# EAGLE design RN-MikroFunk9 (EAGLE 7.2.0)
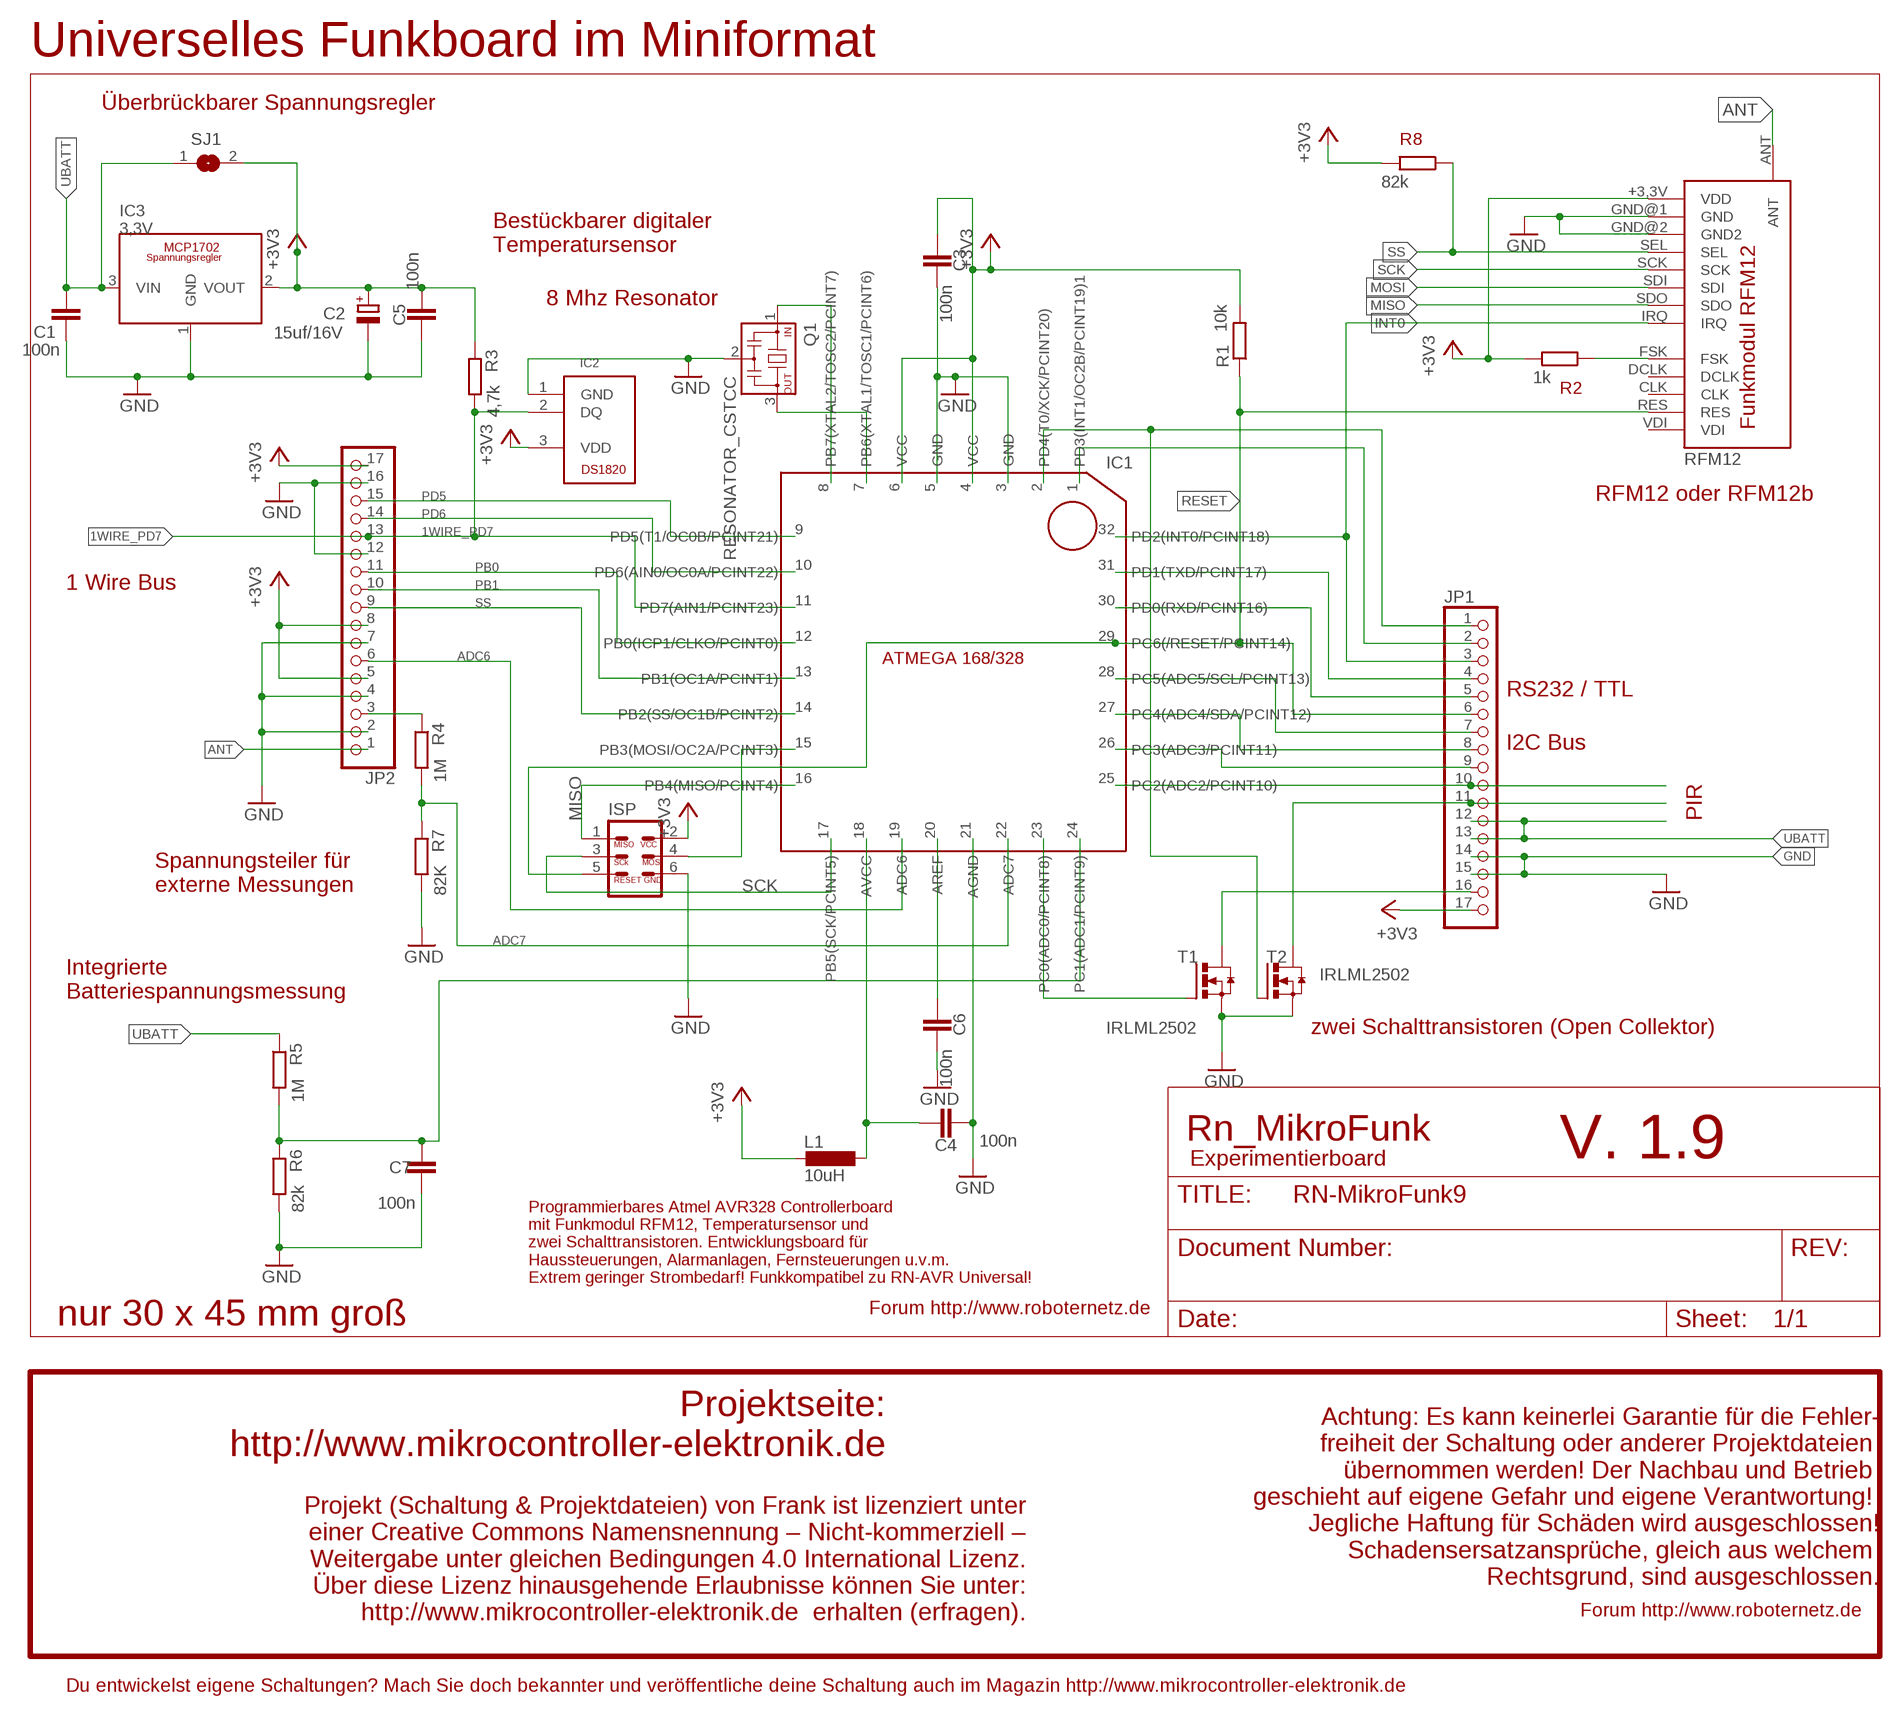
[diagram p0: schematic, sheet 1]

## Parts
C1  100n  C-EUC1206  [C1206]
C2  15uf/16V  CPOL-EUSMCC  [SMC_C]
C3  100n  C-EUC1206  [C1206]
C4  100n  C-EUC1206  [C1206]
C5  100n  C-EUC1206  [C1206]
C6  100n  C-EUC1206  [C1206]
C7  100n  C-EUC1206  [C1206]
IC1  ATMEGA168/328_SMD_PINANSICHT  [TQFP32-08]
IC2  DS1820  [TO92-]
IC3  3,3V  MCP1702SOT23  [SOT23]
ISP  ISP6  [ISP6DICK]
JP1  PINHD-1X17  [1X17]
JP2  PINHD-1X17  [1X17]
L1  10uH  L-SMD-1206  [L1206]
Q1  RESONATOR_CSTCC  [RESONATOR_CSTCC]
R1  10k  R-EU_M1206  [M1206]
R2  1k  R-EU_M1206  [M1206]
R3  4,7k  R-EU_M1206  [M1206]
R4  1M  R-EU_M1206  [M1206]
R5  1M  R-EU_M1206  [M1206]
R6  82k  R-EU_M1206  [M1206]
R7  82K  R-EU_M1206  [M1206]
R8  82k  R-EU_M1206  [M1206]
RFM12  RFM12  [RFM12_SMD]
SJ1  SJ  [SJ]
T1  IRLML2502  [MICRO3]
T2  IRLML2502  [MICRO3]

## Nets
1WIRE_PD7: IC1.11(PD7(AIN1/PCINT23)) IC2.2(DQ) JP2.13 R3.2
+3V3 [Power]: C2.+ C3.2 C5.1 IC1.4(VCC) IC1.6(VCC) IC2.3(VDD) IC3.2(VOUT) ISP.2 JP1.17 JP2.5 JP2.8 JP2.17 L1.2 R1.2 R2.2 R3.1 R8.2 RFM12.+3,3V(VDD) SJ1.2
ADC2: IC1.25(PC2(ADC2/PCINT10)) JP1.10
ADC3: IC1.26(PC3(ADC3/PCINT11)) JP1.9
ADC4: IC1.27(PC4(ADC4/SDA/PCINT12)) JP1.8
ADC5: IC1.28(PC5(ADC5/SCL/PCINT13)) JP1.7
ADC6: IC1.19(ADC6) JP2.6
ADC7: IC1.22(ADC7) R4.2 R7.1
ANT: JP2.1 RFM12.ANT
GND [Power]: C1.1 C2.- C3.1 C4.1 C5.2 C6.1 C7.1 IC1.3(GND) IC1.5(GND) IC1.21(AGND) IC2.1(GND) IC3.1(GND) ISP.6 JP1.14 JP1.15 JP2.2 JP2.4 JP2.7 JP2.12 JP2.16 Q1.2 R6.2 R7.2 RFM12.GND@1(GND) RFM12.GND@2(GND2) T1.2(S) T2.2(S)
INT0: IC1.32(PD2(INT0/PCINT18)) JP1.3 RFM12.IRQ
INT1: IC1.1(PD3(INT1/OC2B/PCINT19)1) JP1.2
MISO: IC1.16(PB4(MISO/PCINT4)) ISP.1 RFM12.SDO
MOSI: IC1.15(PB3(MOSI/OC2A/PCINT3)) ISP.4 RFM12.SDI
N$2: IC1.7(PB6(XTAL1/TOSC1/PCINT6)) Q1.3
N$3: C4.2 IC1.18(AVCC) L1.1
N$5: IC1.8(PB7(XTAL2/TOSC2/PCINT7)) Q1.1
N$6: C6.2 IC1.20(AREF)
N$8: R2.1 RFM12.FSK
N$10 [Power]: IC1.23(PC0(ADC0/PCINT8)) T1.1(G)
N$18: JP2.3 R4.1
N$20: C7.2 IC1.24(PC1(ADC1/PCINT9)) R5.2 R6.1
PB0: IC1.12(PB0(ICP1/CLKO/PCINT0)) JP2.11
PB1: IC1.13(PB1(OC1A/PCINT1)) JP2.10
PD1: IC1.2(PD4(T0/XCK/PCINT20)) JP1.1 T2.1(G)
PD5: IC1.9(PD5(T1/OC0B/PCINT21)) JP2.15
PD6: IC1.10(PD6(AIN0/OC0A/PCINT22)) JP2.14
RESET: IC1.29(PC6(/RESET/PCINT14)) ISP.5 JP1.6 R1.1 RFM12.RES
RXD: IC1.30(PD0(RXD/PCINT16)) JP1.5
SCK: IC1.17(PB5(SCK/PCINT5)) ISP.3 RFM12.SCK
SS: IC1.14(PB2(SS/OC1B/PCINT2)) JP2.9 R8.1 RFM12.SEL
T1 [Power]: JP1.16 T1.3(D)
T2 [Power]: JP1.11 T2.3(D)
TXD: IC1.31(PD1(TXD/PCINT17)) JP1.4
UBATT [Power]: C1.2 IC3.3(VIN) JP1.12 JP1.13 R5.1 SJ1.1
Unconnected: RFM12.CLK RFM12.DCLK RFM12.VDI

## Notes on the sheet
- Universelles Funkboard im Miniformat
- Überbrückbarer Spannungsregler
- R8
- Bestückbarer digitaler
  Temperatursensor
- 8 Mhz Resonator
- R2
- RFM12 oder RFM12b
- 1 Wire Bus
- RS232 / TTL
- I2C Bus
- PIR
- Spannungsteiler für
  externe Messungen
- Integrierte 
  Batteriespannungsmessung
- zwei Schalttransistoren (Open Collektor)
- Rn_MikroFunk
- V. 1.9
- Experimentierboard
- Programmierbares Atmel AVR328 Controllerboard
  mit Funkmodul RFM12, Temperatursensor und
  zwei Schalttransistoren. Entwicklungsboard für 
  Haussteuerungen, Alarmanlagen, Fernsteuerungen u.v.m.
  Extrem geringer Strombedarf! Funkkompatibel zu RN-AVR Universal!
- Forum http://www.roboternetz.de
- nur 30 x 45 mm groß
- Projektseite:
  http://www.mikrocontroller-elektronik.de
- Achtung: Es kann keinerlei Garantie für die Fehler-
  freiheit der Schaltung oder anderer Projektdateien 
  übernommen werden! Der Nachbau und Betrieb 
  geschieht auf eigene Gefahr und eigene Verantwortung! 
  Jegliche Haftung für Schäden wird ausgeschlossen!
  Schadensersatzansprüche, gleich aus welchem 
  Rechtsgrund, sind ausgeschlossen.
- Projekt (Schaltung & Projektdateien) von Frank ist lizenziert unter
  einer Creative Commons Namensnennung – Nicht-kommerziell –
  Weitergabe unter gleichen Bedingungen 4.0 International Lizenz.
  Über diese Lizenz hinausgehende Erlaubnisse können Sie unter:
  http://www.mikrocontroller-elektronik.de  erhalten (erfragen).
- Forum http://www.roboternetz.de
- Du entwickelst eigene Schaltungen? Mach Sie doch bekannter und veröffentliche deine Schaltung auch im Magazin http://www.mikrocontroller-elektronik.de

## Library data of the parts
C1 C3-C7 = rcl:C-EU: CAPACITOR, European symbol
C2 = rcl:CPOL-EU: POLARIZED CAPACITOR, European symbol
IC1 = RoboterNetzNeu:ATMEGA168/328_SMD_PINANSICHT: ATMEGA 168/328 etc.SMD Pinansicht (robotikhardware.de)
IC2 = RoboterNetzNeu:DS1820: Temperatursensor Dallas DS1820 oder DS18S20 etc. (Bezug Robotikhardware.de)
IC3 = RoboterNetzNeu:MCP1702: MCP 1702-3302 :: Positiv Spannungsregler 3,3V / 200 mA / Low-Current 2µA / max. 13,2 V
ISP = RoboterNetzNeu:ISP6: 6 poliger Standard ISP Stecker (Bezug: 10 auf 6 Adapter bei Robotikhardware.de)
JP1 JP2 = pinhead:PINHD-1X17: PIN HEADER
L1 = RoboterNetzNeu:L-SMD-1206: L-1206F 10µ :: SMD-Induktivität, 1206, Ferrit, 10µ Reichelt Best.nr L-1206F 10µ
Q1 = RoboterNetzNeu:RESONATOR_CSTCC: Resonator(z.B. CSTCC8.00 bei Reichelt oder Robotikhardware.de)
R1-R8 = rcl:R-EU_: RESISTOR, European symbol
RFM12 = RoboterNetzNeu:RFM12: Funkmodul RFM12 (siehe roboternetz.de / robotikhardware.de)
SJ1 = jumper:SJ: SMD solder JUMPER
T1 T2 = RoboterNetzNeu:IRLML2502: HEXFET IRLML2502 20V/4,2A

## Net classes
0 default: width 0.254 mm
1 Power: width 0.406 mm

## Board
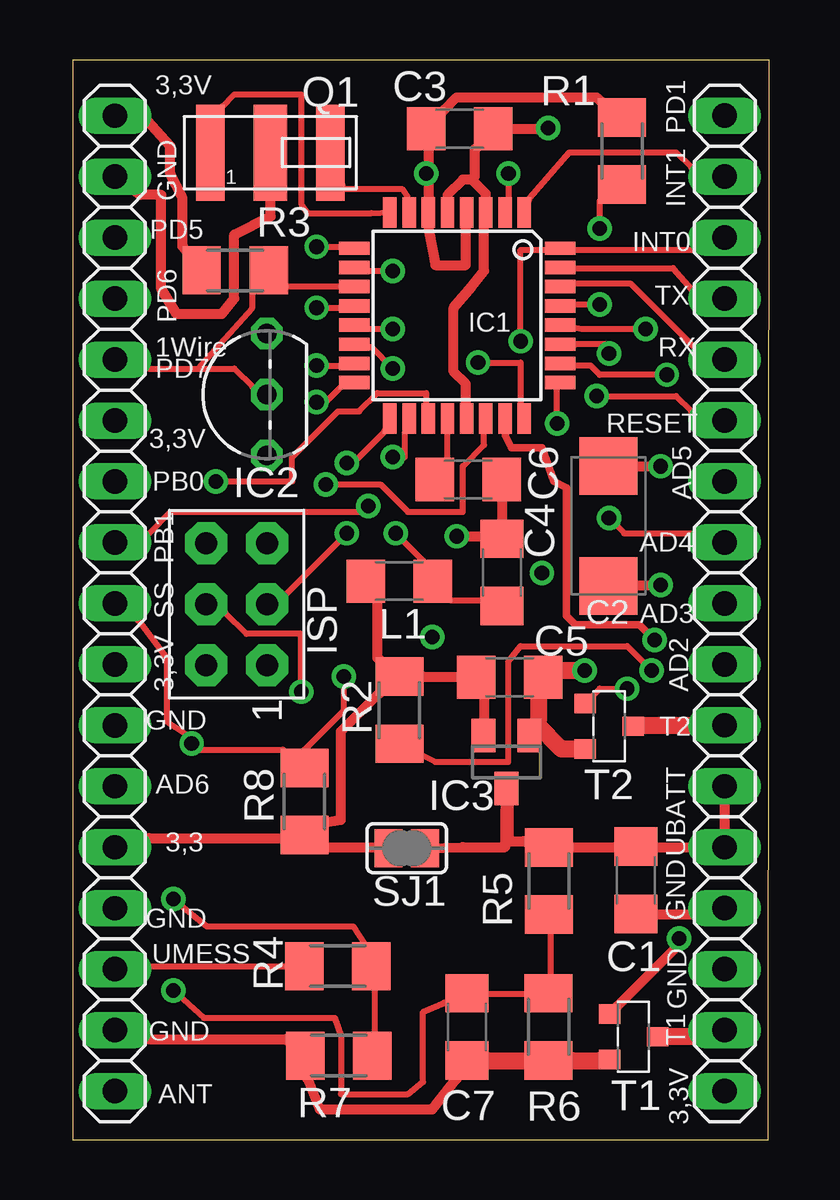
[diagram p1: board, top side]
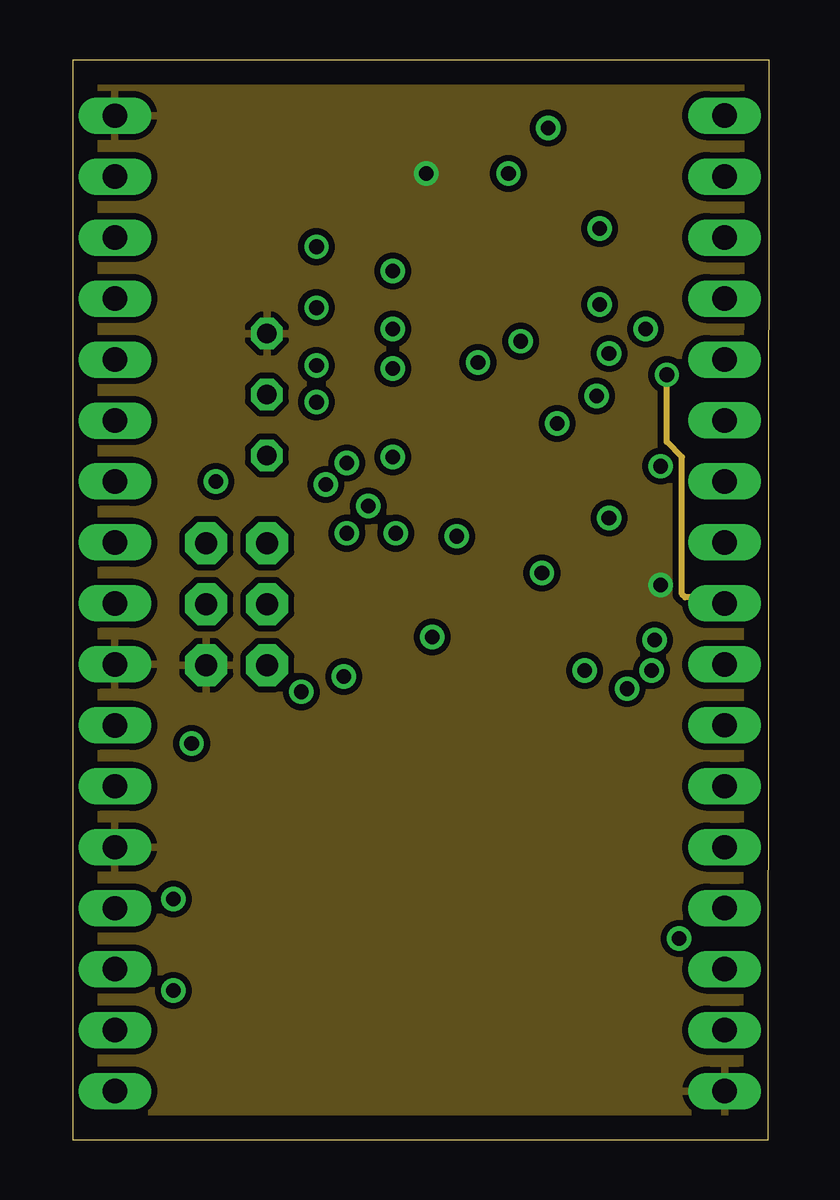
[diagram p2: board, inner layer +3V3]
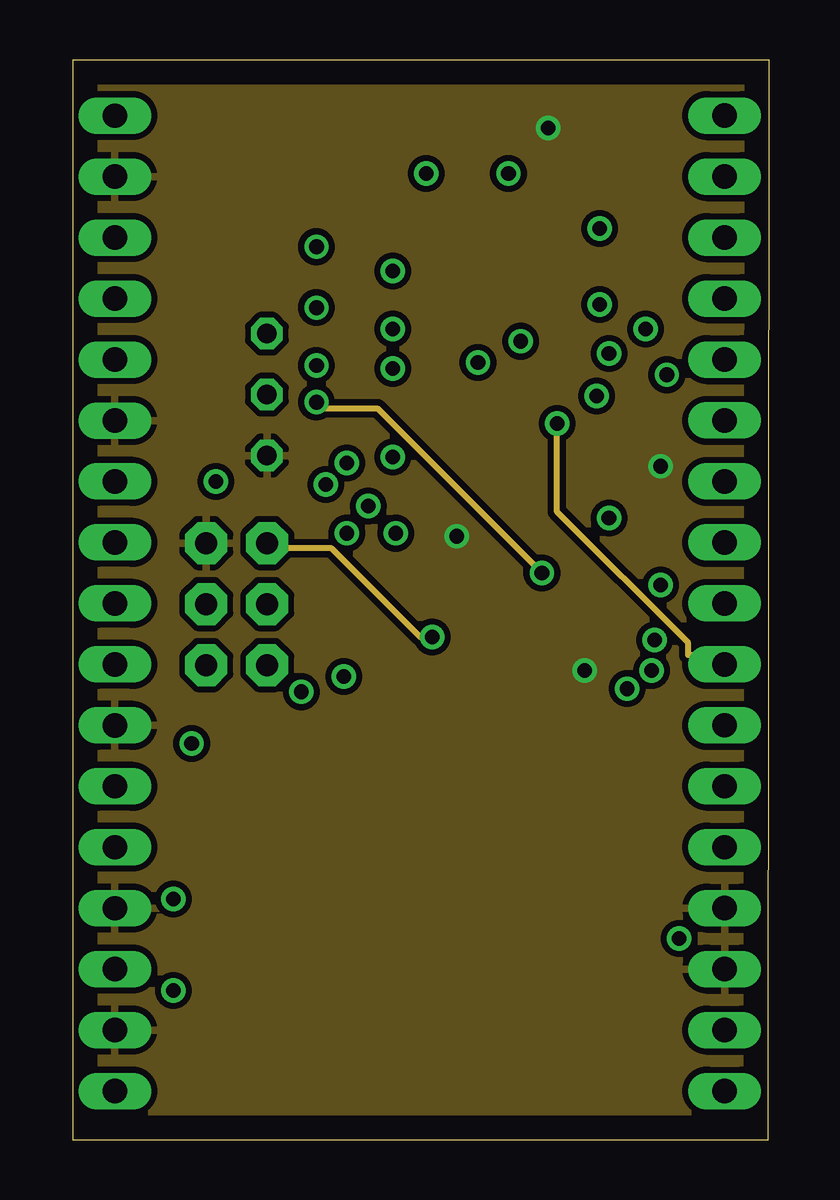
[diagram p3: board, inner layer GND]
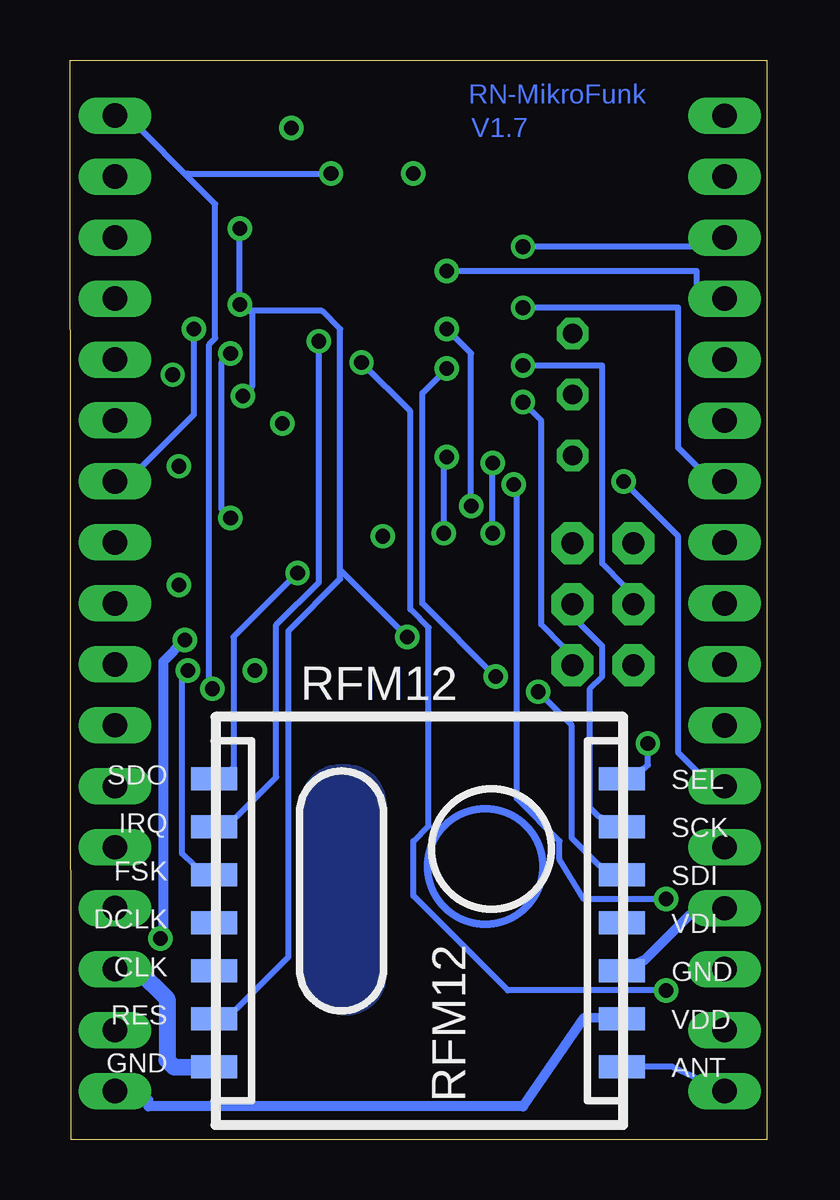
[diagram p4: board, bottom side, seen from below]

Size 29.03 x 44.99 mm. Coordinates in mm from the lower left corner, seen from the top.
Outline: 0,0 29,0 29.03,44.99 0,44.99 0,0
Copper layers (1+2*15+16): Top 0.035mm / dielectric 0.5mm / +3V3 0.035mm / dielectric 0.5mm / GND 0.035mm / dielectric 0.5mm / Bottom 0.035mm
Design rules "default *": minimum track width 8mil, minimum drill 24mil, track to track 8mil, track to pad 8mil, pad to pad 8mil, via to via 8mil, smd to smd 8mil, copper to edge 40mil, drill to drill 8mil, minimum pad ring 10mil, minimum via ring 8mil, stop-mask expansion 4mil, vias tented up to drill 0mil, thermal gap 10mil

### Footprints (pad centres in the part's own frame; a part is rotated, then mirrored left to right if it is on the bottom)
C1206 = smd 1.6 x 1.8: 1 -1.4,0; 2 1.4,0
SMC_C = smd 2.4 x 2.4: + -2.5,0; - 2.5,0
TQFP32-08 = smd 1.27 x 0.559: 1 -4.293,2.8; 2 -4.293,2; 3 -4.293,1.2; 4 -4.293,0.4; 5 -4.293,-0.4; 6 -4.293,-1.2; 7 -4.293,-2; 8 -4.293,-2.8; 17 4.293,-2.8; 18 4.293,-2; 19 4.293,-1.2; 20 4.293,-0.4; 21 4.293,0.4; 22 4.293,1.2; 23 4.293,2; 24 4.293,2.8 | smd 0.559 x 1.27: 9 -2.8,-4.293; 10 -2,-4.293; 11 -1.2,-4.293; 12 -0.4,-4.293; 13 0.4,-4.293; 14 1.2,-4.293; 15 2,-4.293; 16 2.8,-4.293; 25 2.8,4.293; 26 2,4.293; 27 1.2,4.293; 28 0.4,4.293; 29 -0.4,4.293; 30 -1.2,4.293; 31 -2,4.293; 32 -2.8,4.293
TO92- = drill 0.813 octagon: 1 -2.54,0; 2 0,0; 3 2.54,0
SOT23 = smd 1 x 1.4: 1 -0.95,-1.1; 2 0.95,-1.1; 3 0,1.1
ISP6DICK = drill 0.914 pad 1.75 octagon: 1 -2.54,-1.27; 2 -2.54,1.27; 3 0,-1.27; 4 0,1.27; 5 2.54,-1.27; 6 2.54,1.27
1X17 = drill 1.016 long: 1 -20.32,0; 2 -17.78,0; 3 -15.24,0; 4 -12.7,0; 5 -10.16,0; 6 -7.62,0; 7 -5.08,0; 8 -2.54,0; 9 0,0; 10 2.54,0; 11 5.08,0; 12 7.62,0; 13 10.16,0; 14 12.7,0; 15 15.24,0; 16 17.78,0; 17 20.32,0
L1206 = smd 1.6 x 1.8: 1 -1.4,0; 2 1.4,0
RESONATOR_CSTCC = smd 1.2 x 4: 1 2.5,0; 3 -2.5,0 | smd 1.4 x 4: 2 0,0
M1206 = smd 1.6 x 2: 1 -1.4,0; 2 1.4,0
RFM12_SMD = smd 0.965 x 1.93: +3,3V 0,5.5; ANT 2,5.5; CLK -2,-11.5; DCLK -4,-11.5; FSK -6,-11.5; GND@1 2,-11.5; GND@2 -2,5.5; IRQ -8,-11.5; RES 0,-11.5; SCK -8,5.5; SDI -6,5.5; SDO -10,-11.5; SEL -10,5.5; VDI -4,5.5
SJ = smd 1.168 x 1.6: 1 -0.762,0; 2 0.762,0
MICRO3 = smd 0.8 x 0.9: 1 -0.95,-1; 2 0.95,-1; 3 0,1

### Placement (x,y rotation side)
C1  23.47,10.81 90 top
C2  22.33,25.58 90 top
C3  16.13,42.13 180 top
C4  17.89,23.64 270 top
C5  18.21,19.27 0 top
C6  16.48,27.51 180 top
C7  16.43,4.71 90 top
IC1  16.02,34.35 270 top
IC2  8.09,31.05 90 top
IC3  18.08,15.74 180 top
ISP  6.83,22.32 90 top
JP1  27.18,22.35 270 top
JP2  1.75,22.35 90 top
L1  13.61,23.28 180 top
Q1  8.24,41.14 180 top
R1  22.9,41.2 90 top
R2  13.61,17.9 90 top
R3  6.77,36.23 0 top
R4  11.05,7.24 0 top
R5  19.85,10.78 270 top
R6  19.84,4.71 270 top
R7  11.09,3.51 180 top
R8  9.65,14.1 270 top
RFM12  11.54,5.04 270 bottom
SJ1  13.92,12.15 180 top
T1  23.37,4.3 270 top
T2  22.36,17.23 270 top

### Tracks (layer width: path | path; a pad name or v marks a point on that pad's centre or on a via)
1WIRE_PD7
  Top 0.254: IC1.11 11.18,35.56 8.89,35.56 R3.2 7.49,35.31 7.49,34.67 5.21,32.13 | 5.21,32.13 3.17,32.13 JP2.13 | 5.21,32.13 6.73,32.13 7.49,31.37 IC2.2
+3V3  (via drill 0.61)
  Top 0.406: 14.86,40.26 14.86,41.27 C3.2 15.49,42.93 16,43.43 21.84,43.43 21.97,43.31 R1.2 | 14.86,40.26 14.86,39.24 IC1.6 14.86,38.1 14.86,37.85 15.11,36.45 16.38,36.45 16.38,38.1 IC1.4 | IC3.2 17.14,17.53 17.14,18.41 C5.1 16.13,19.3 14.61,19.3 R2.2 | L1.2 12.7,22.48 12.7,20.07 R2.2 | SJ1.2 12.7,12.19 10.54,12.19 R8.2 | R3.1 4.57,37.21 4.57,39.24 4.06,40.26 4.06,41.4 2.92,42.67 JP2.17 | v24.51,23.11 23.5,23.11 C2.+ | R8.2 8.76,12.57 3.17,12.57 JP2.5 | R2.2 12.7,18.54 11.18,17.02 11.18,13.34 10.41,13.21 R8.2 | 14.86,40.26 v14.73,40.26
  Bottom 0.406: RFM12.+3,3V 7.62,5.08 10.16,1.4 25.78,1.4 25.78,1.65 JP1.17
  pour +3V3 (isolate 0.254): 0.25,0.25 28.75,0.25 28.75,44.75 0.25,44.75
ADC2  (via drill 0.61)
  Top 0.254: v20.19,29.84 20.19,31.37 IC1.25
  GND 0.254: v20.19,29.84 20.19,26.16 25.65,20.7 25.65,20.19 26.54,20.19 JP1.10
ADC3  (via drill 0.61)
  Top 0.254: v24.77,31.88 21.97,31.88 21.59,32.26 20.83,32.26 IC1.26
  +3V3 0.254: v24.77,31.88 24.77,29.08 25.4,28.45 25.4,22.73 25.53,22.61 26.54,22.61 JP1.9
ADC4  (via drill 0.61)
  Top 0.254: v22.35,32.77 22.23,33.15 20.95,33.15 IC1.27 | v22.35,25.91 22.99,25.27 25.78,25.27 JP1.8
  Bottom 0.254: v22.35,32.77 22.73,32.38 22.73,26.29 v22.35,25.91
ADC5  (via drill 0.61)
  Top 0.254: v23.88,33.78 21.21,33.78 IC1.28
  Bottom 0.254: v23.88,33.78 23.88,30.23 26.04,28.07 JP1.7
ADC6  (via drill 0.61)
  Top 0.254: v5.97,27.43 9.14,27.43 9.14,28.45 11.05,30.35 11.94,30.35 12.7,31.11 14.73,31.11 14.73,30.61 IC1.19
  Bottom 0.254: v5.97,27.43 3.68,25.15 3.68,16.13 2.92,15.37 JP2.6
ADC7  (via drill 0.61)
  Top 0.254: v10.54,27.3 12.83,27.3 13.97,26.16 16.26,26.16 16.26,28.07 17.14,28.96 17.14,29.46 IC1.22 | v4.19,10.03 5.59,8.89 11.68,8.89 12.19,8.13 R4.2 12.57,6.35 12.57,4.45 R7.1
  Bottom 0.254: v10.54,27.3 10.41,27.18 10.41,14.22 8.64,12.45 8.64,11.68 7.62,10.03 v4.19,10.03
ANT
  Bottom 0.254: RFM12.ANT 5.08,3.05 3.94,3.05 JP2.1
GND  (via drill 0.61)
  Top 0.406: IC1.21 16.38,30.61 16.38,31.5 15.88,32 15.88,34.67 16.64,35.56 17.14,36.2 17.14,38.1 IC1.3 17.22,39.42 16.64,40.01 | 21.97,3.3 T1.2 | 20.83,3.3 R6.2 18.92,3.3 | 17.27,3.3 C7.1 16,2.54 14.99,1.27 10.29,1.27 9.78,2.54 R7.2 8.89,4.19 3.17,4.19 JP2.2 | 19.43,18.41 C5.2 20.32,19.56 | IC3.1 19.28,17.27 19.43,17.53 | C6.1 17.91,26.67 17.91,25.78 C4.1 17.02,25.15 v16,25.15 | C1.1 24.26,9.4 25.78,9.4 JP1.14 | v24.51,28.07 23.5,28.07 C2.- | Q1.2 8.26,39.24 8.26,38.48 6.73,37.72 6.73,35.05 6.22,34.42 4.32,34.42 3.68,35.43 3.68,39.37 2.79,39.37 JP2.16 | v19.81,42.16 19.81,42.13 C3.1 16.76,41.27 16.76,40.13 16.64,40.01 | 16.64,40.01 16.26,40.01 15.62,39.37 IC1.5
  Top 0.7: 20.83,3.3 21.97,3.3 | 17.27,3.3 18.92,3.3 | 19.43,17.53 19.43,18.41 | 20.32,19.56 v21.34,19.56 | T2.2 20.38,16.27 19.38,17.27 19.28,17.27
  Bottom 0.406: RFM12.GND@2 5.08,7.49 3.17,9.4 JP2.4
  Bottom 0.7: JP1.15 26.24,7.11 25,5.88 25,3.33 24.7,3.02 RFM12.GND@1
  pour GND (isolate 0.254): 0.25,0.25 0.25,44.5 28.75,44.5 28.75,0.25
INT0  (via drill 0.61)
  Top 0.254: JP1.3 25.91,37.08 20.83,37.08 IC1.32 19.68,37.08 18.67,37.08 v18.67,33.27
  Bottom 0.254: v18.67,33.27 18.67,23.24 20.45,21.46 20.45,15.11 22.1,13.46 RFM12.IRQ
INT1
  Top 0.254: IC1.1 19.05,39.24 20.7,41.15 25.15,41.15 25.78,40.51 JP1.2
MISO  (via drill 0.61)
  Top 0.254: v10.16,30.73 10.54,30.73 11.18,31.37 IC1.16
  GND 0.254: v19.56,23.62 12.7,30.48 10.54,30.48 v10.16,30.73
  Bottom 0.254: v10.16,30.73 9.4,29.97 9.4,21.46 8.51,20.57 ISP.1 | v19.56,23.62 22.23,20.95 22.23,15.49 RFM12.SDO
MOSI  (via drill 0.61)
  Top 0.254: v10.16,32.26 11.18,32.26 IC1.15 | v9.53,18.67 9.53,21.08 7.24,21.08 6.35,21.97 ISP.4
  Bottom 0.254: v10.16,32.26 6.86,32.26 6.86,24 5.97,23.11 ISP.4 | v9.53,18.67 8.13,17.27 8.13,12.57 6.99,11.43 RFM12.SDI
N$2
  Top 0.254: IC1.7 13.97,39.24 13.72,39.62 11.3,39.62 Q1.3
N$3  (via drill 0.61)
  Top 0.254: v13.34,28.45 13.84,28.45 13.84,29.46 IC1.18 | v13.46,25.27 14.61,24.13 L1.1 15.75,22.48 17.02,22.48 C4.2
  Bottom 0.254: v13.34,28.45 13.46,28.32 v13.46,25.27
N$5
  Top 0.254: IC1.8 12.45,38.61 9.78,38.61 9.53,38.99 9.53,43.56 6.73,43.56 6.22,43.05 Q1.1
N$6
  Top 0.254: IC1.20 15.62,29.46 15.62,28.32 C6.2
N$8  (via drill 0.61)
  Top 0.254: v24.13,19.56 23.11,20.57 18.67,20.57 18.16,19.94 18.16,15.75 15.11,15.75 R2.1
  Bottom 0.254: v24.13,19.56 24.38,19.3 24.38,11.94 23.88,11.43 RFM12.FSK
N$10  (via drill 0.61)
  Top 0.305: v24.26,20.83 23.62,21.46 20.95,21.46 20.57,21.84 20.57,27.18 20.07,27.43 19.56,28.83 18.29,28.83 18.03,29.34 IC1.23
  Top 0.406: v25.27,8.38 25.27,8.13 22.73,5.59 T1.1
  Bottom 0.406: v25.27,8.38 25.15,8.51 25.15,19.94 v24.26,20.83
N$12
  pour Bottom (isolate 0.254): 16,13.72 16,6.86 arc90 17.53,5.33 arc81 19.3,6.86 19.3,13.97 arc90 17.78,15.49 17.53,15.49 arc90 16,13.97
N$18
  Top 0.254: R4.1 3.17,7.24 JP2.3
N$20  (via drill 0.61)
  Top 0.254: v16.89,32.38 18.67,32.38 18.67,30.61 IC1.24 | v4.19,6.22 5.46,5.08 10.92,5.08 11.18,4.32 11.18,1.91 13.97,1.91 14.61,2.41 14.61,5.33 15.49,5.71 C7.2 17.27,6.1 18.92,6.1 R6.1 19.94,6.86 19.94,8.64 R5.2
  Bottom 0.254: v16.89,32.38 14.86,30.35 14.86,22.1 14.1,21.34 14.1,13.08 14.73,12.45 14.73,10.16 10.79,6.22 v4.19,6.22
PB0  (via drill 0.61)
  Top 0.254: v10.16,34.67 11.18,34.67 IC1.12
  Bottom 0.254: v10.16,34.67 3.68,34.67 3.68,28.83 2.92,28.07 JP2.11
PB1  (via drill 0.61)
  Top 0.254: v13.34,33.78 12.32,33.78 IC1.13 | v12.32,26.42 12.06,26.16 4.06,26.16 3.17,25.27 JP2.10
  Bottom 0.254: v13.34,33.78 12.32,32.77 v12.32,26.42
PD1  (via drill 0.61)
  Top 0.254: v23.11,18.8 21.97,18.8 21.72,18.54 T2.1 | v18.16,40.26 18.16,39.24 IC1.2
  Bottom 0.254: v23.11,18.8 23.24,18.92 23.24,33.15 22.99,33.4 22.99,38.99 24.19,40.2 | 24.19,40.2 26.04,42.04 JP1.1 | v18.16,40.26 24.13,40.26 24.19,40.2
PD5  (via drill 0.61)
  Top 0.254: v10.16,37.21 11.18,37.21 IC1.9
  Bottom 0.254: v10.16,37.21 3.17,37.21 JP2.15
PD6  (via drill 0.61)
  Top 0.254: v13.34,36.2 12.32,36.2 IC1.10
  Bottom 0.254: v13.34,36.2 2.92,36.2 2.92,35.69 JP2.14
RESET  (via drill 0.61)
  Top 0.254: v21.97,34.8 20.83,34.8 IC1.29 | v21.97,37.97 21.97,39.12 R1.1 | v21.84,30.99 25.15,30.99 25.78,30.35 JP1.6
  GND 0.254: v14.99,20.95 14.48,20.95 10.79,24.64 8.76,24.64 ISP.5
  Bottom 0.254: v21.97,37.97 v21.97,34.8 21.59,34.54 21.46,34.54 | 17.78,23.75 17.78,33.78 18.54,34.54 21.46,34.54 | 17.78,23.75 17.78,23.37 19.94,21.21 19.94,7.62 22.1,5.46 RFM12.RES | v21.84,30.99 21.46,31.37 21.46,34.54 | 17.78,23.75 v14.99,20.95
RXD
  Top 0.254: IC1.30 20.83,35.69 23.24,35.69 25.91,33.02 JP1.5
SCK  (via drill 0.61)
  Top 0.254: v11.43,28.19 11.68,28.19 12.95,29.46 IC1.17 | v11.43,25.27 8.89,22.73 ISP.3
  Bottom 0.254: v11.43,25.27 v11.43,28.19 | RFM12.SCK 6.99,13.46 7.37,13.84 7.37,18.8 6.86,19.3 6.86,20.57 7.75,21.46 ISP.3
SS  (via drill 0.61)
  Top 0.254: v13.34,32.13 12.45,33.02 12.32,33.02 IC1.14 | v11.3,19.3 11.3,17.91 9.65,16.26 R8.1 8.76,16.26 5.21,16.26 v4.95,16.51 4.7,16.89 3.94,17.4 3.94,20.07 2.79,21.59 JP2.9
  Bottom 0.254: v13.34,32.13 14.35,31.11 14.35,22.35 v11.3,19.3 | v4.95,16.51 4.95,15.62 5.08,15.49 RFM12.SEL
T1
  Top 0.406: T1.3 24.77,4.32
  Top 0.7: JP1.16 26.9,4.3 T1.3
T2
  Top 0.406: T2.3 23.75,17.27
  Top 0.7: 23.75,17.27 JP1.11
TXD
  Top 0.254: IC1.31 20.83,36.32 25.02,36.32 25.78,35.43 JP1.4
UBATT
  Top 0.406: SJ1.1 16.26,12.19 18.03,12.19 18.03,13.46 IC3.3 18.16,13.84 18.16,12.45 18.8,12.45 R5.1 20.83,12.19 22.61,12.19 C1.2 24.26,12.19 JP1.13 JP1.12
(copper drawn outside any net)
  shapes: Bottom circle x1

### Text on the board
Bottom: RN-MikroFunk | V1.7
tPlace: 3,3V | PD1 | GND | INT1 | PD5 | INT0 | TX | PD6 | 1Wire | RX | PD7 | 3,3V | RESET | PB0 | AD5 | AD4 | PB1 | SS | AD3 | 3,3V | AD2 | GND | T2 | AD6 | 3,3 | UBATT | GND | GND | GND | UMESS | GND | T1 | ANT | 3,3V
Document: RN-MikroFunk / Modul mit AtMega328 und RFM12b / / Hauptaufgabengebiet: / Funk Aktoren / Funk Sensoren / Alarmanlage / Fernsteuerung | V. 1.9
